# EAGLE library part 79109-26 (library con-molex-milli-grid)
RECEPTACAL
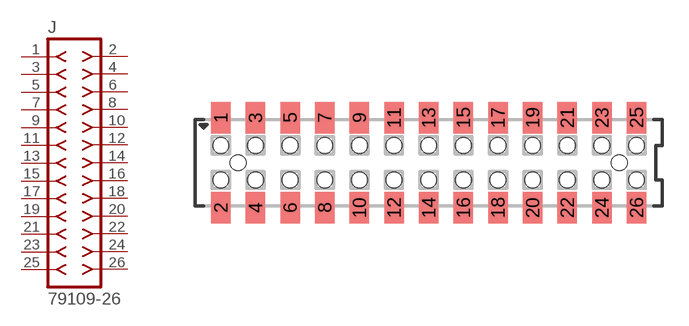
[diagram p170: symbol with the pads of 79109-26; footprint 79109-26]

Designator prefix J

## 79109-26  [79109-26]
1  1  pas
2  2  pas
3  3  pas
4  4  pas
5  5  pas
6  6  pas
7  7  pas
8  8  pas
9  9  pas
10  10  pas
11  11  pas
12  12  pas
13  13  pas
14  14  pas
15  15  pas
16  16  pas
17  17  pas
18  18  pas
19  19  pas
20  20  pas
21  21  pas
22  22  pas
23  23  pas
24  24  pas
25  25  pas
26  26  pas

## Footprint 79109-26 (pad centres in mm)
RECEPTACAL SMD Dual Row, Vertical, Pass-Thru
smd 1.12 x 1.83: 1 -12,2.6; 2 -12,-2.6; 3 -10,2.6; 4 -10,-2.6; 5 -8,2.6; 6 -8,-2.6; 7 -6,2.6; 8 -6,-2.6; 9 -4,2.6; 10 -4,-2.6; 11 -2,2.6; 12 -2,-2.6; 13 0,2.6; 14 0,-2.6; 15 2,2.6; 16 2,-2.6; 17 4,2.6; 18 4,-2.6; 19 6,2.6; 20 6,-2.6; 21 8,2.6; 22 8,-2.6; 23 10,2.6; 24 10,-2.6; 25 12,2.6; 26 12,-2.6
hole 0.914 at -11,0
hole 0.914 at -12,1
hole 0.914 at -12,-1
hole 0.914 at -10,-1
hole 0.914 at -10,1
hole 0.914 at -8,-1
hole 0.914 at -8,1
hole 0.914 at 11,0
hole 0.914 at -6,1
hole 0.914 at -6,-1
hole 0.914 at -4,1
hole 0.914 at -4,-1
hole 0.914 at -2,1
hole 0.914 at -2,-1
hole 0.914 at 0,1
hole 0.914 at 0,-1
hole 0.914 at 2,-1
hole 0.914 at 2,1
hole 0.914 at 4,1
hole 0.914 at 4,-1
hole 0.914 at 6,1
hole 0.914 at 6,-1
hole 0.914 at 8,1
hole 0.914 at 8,-1
hole 0.914 at 10,-1
hole 0.914 at 10,1
hole 0.914 at 12,1
hole 0.914 at 12,-1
